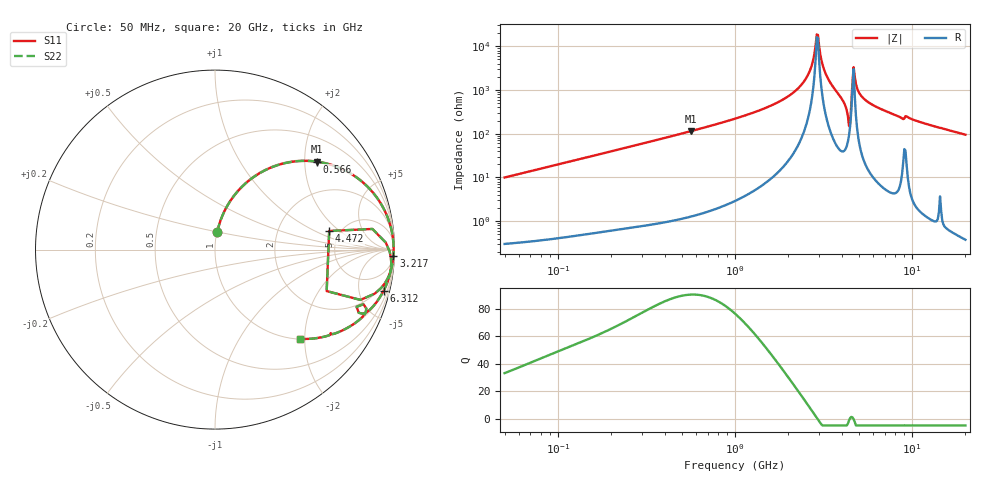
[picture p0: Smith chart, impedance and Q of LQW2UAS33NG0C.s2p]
!Murata Part Number: LQW2UAS33NG0C
!These Parameters are Measured in Series Mode Connection
!  o--[Z]--o
!Port1  Port2
!  o-------o
!Freq. Start=50[MHz] Stop=20[GHz], 401[Steps]
# Hz S RI R 50
!Freq.(Hz) S11(Real) S11(Imag) S21(Real) S21(Imag) S12(Real) S12(Imag) S22(Real) S22(Imag)
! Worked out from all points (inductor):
!   401 points, 50 MHz to 20 GHz, reference 50 ohm
!   read as one part in series: L = 31.6 nH near 51.52 MHz
!   highest Q = 90.2 at 566 MHz (marker M1), where L = 32.3 nH
!   self-resonance near 2.896 GHz
!   S11 on the Smith chart (normalised r, x): 50 MHz: 1.01, +0.20; 566 MHz: 1.03, +2.30; 3.217 GHz: 8, -52; 4.472 GHz: 4.09, +1.45; 6.312 GHz: 1.16, -8.15; 20 GHz: 1.01, -1.90
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5e7  0.0127 0.0978  0.9873 -0.0978  0.9873 -0.0978  0.0127 0.0978
1.364002e8  0.0715 0.2489  0.9285 -0.2489  0.9285 -0.2489  0.0715 0.2489
3.721004e8  0.3557 0.4728  0.6443 -0.4728  0.6443 -0.4728  0.3557 0.4728
5.659842e8  0.5681 0.4898  0.4319 -0.4898  0.4319 -0.4898  0.5681 0.4898
1e9  0.826 0.3726  0.174 -0.3726  0.174 -0.3726  0.826 0.3726
1.521052e9  0.938 0.2315  0.062 -0.2315  0.062 -0.2315  0.938 0.2315
2.05233e9  0.9792 0.1259  0.0208 -0.1259  0.0208 -0.1259  0.9792 0.1259
2.456456e9  0.9915 0.0623  0.00846 -0.0623  0.00846 -0.0623  0.9915 0.0623
2.728004e9  0.9948 0.0247  0.00518 -0.0247  0.00518 -0.0247  0.9948 0.0247
2.853386e9  0.9953 0.00822  0.00467 -0.00822  0.00467 -0.00822  0.9953 0.00822
2.940159e9  0.9954 -0.0029  0.00464 0.0029  0.00464 0.0029  0.9954 -0.0029
3.216634e9  0.9938 -0.0374  0.00624 0.0374  0.00624 0.0374  0.9938 -0.0374
4.087748e9  0.9565 -0.1713  0.0435 0.1713  0.0435 0.1713  0.9565 -0.1713
4.275624e9  0.8905 -0.2452  0.1095 0.2452  0.1095 0.2452  0.8905 -0.2452
4.34015e9  0.8104 -0.2804  0.1896 0.2804  0.1896 0.2804  0.8104 -0.2804
4.472136e9  0.6363 0.1037  0.3637 -0.1037  0.3637 -0.1037  0.6363 0.1037
4.608136e9  0.952 0.0387  0.048 -0.0387  0.048 -0.0387  0.952 0.0387
4.748272e9  0.9801 -0.0455  0.0199 0.0455  0.0199 0.0455  0.9801 -0.0455
5.194772e9  0.9743 -0.1362  0.0257 0.1362  0.0257 0.1362  0.9743 -0.1362
6.311513e9  0.9392 -0.2294  0.0608 0.2294  0.0608 0.2294  0.9392 -0.2294
7.442007e9  0.8987 -0.2943  0.1013 0.2943  0.1013 0.2943  0.8987 -0.2943
2e10  0.4747 -0.4974  0.5253 0.4974  0.5253 0.4974  0.4747 -0.4974
